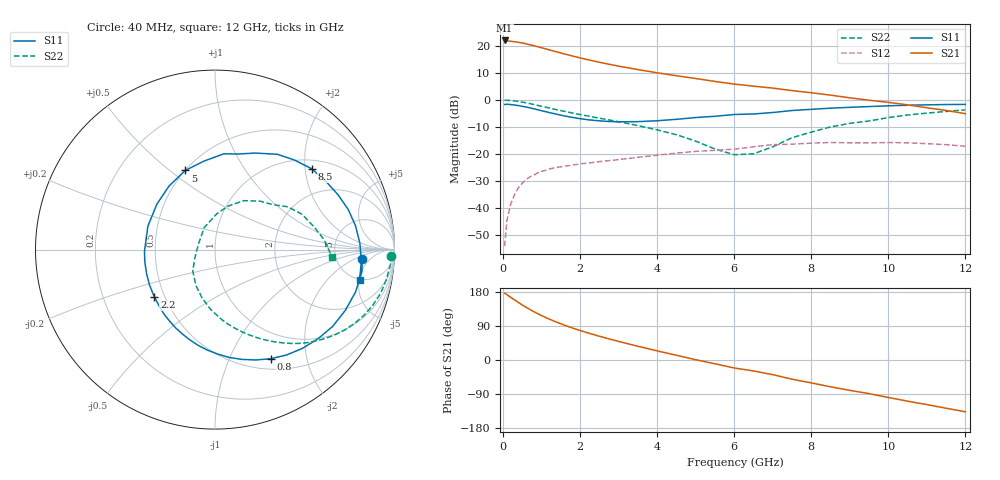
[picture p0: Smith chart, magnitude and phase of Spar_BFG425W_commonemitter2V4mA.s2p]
! Filename: 24bfg425.001
! BFG425W Field C1
! V1=8.240E-001V,V2=2.000E+000V, I1=5.227E-005A, I2=4.000E-003A
# GHz  S  MA  R 50
!  S11  S21  S12  S22
!Freq(GHz)  Mag  Ang  Mag  Ang  Mag  Ang  Mag  Ang
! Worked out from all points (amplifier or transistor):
!   44 points, 40 MHz to 12 GHz, reference 50 ohm
!   highest |S21| = 21.9 dB at 40 MHz (marker M1)
!   |S21| within 3 dB of that: start of sweep to 1.081 GHz
!   unconditionally stable (mu >= 1): 2.635 GHz to end of sweep
!   at 700 MHz: K = 0.29, MSG = 24.3 dB, |S12| = -28.4 dB
!   at 2.4 GHz: K = 0.93, MSG = 18.6 dB, |S12| = -23.0 dB
!   at 12 GHz: K = 1.54, MAG = 1.7 dB, |S12| = -17.1 dB
!   lowest NFmin = 1.00 dB at 900 GHz
!   S11 on the Smith chart (normalised r, x): 40 MHz: 9.30, -2.83; 800 MHz: 0.63, -1.44; 2.2 GHz: 0.44, -0.28; 5 GHz: 0.50, +0.57; 8.5 GHz: 1.22, +2.17; 12 GHz: 4.89, -5.09
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0.04  0.821 -3.5  12.43 176.4  0.002 74.1  0.983 -2.0
0.1  0.828 -8.4  12.17 172.4  0.006 86.0  0.981 -5.0
0.3  0.801 -25.0  11.78 158.6  0.018 74.9  0.954 -14.8
0.5  0.759 -40.9  11.19 145.0  0.029 65.7  0.907 -23.9
0.6  0.735 -48.5  10.77 138.9  0.034 61.4  0.879 -28.0
0.8  0.683 -62.9  9.945 127.6  0.041 54.1  0.819 -35.5
0.9  0.656 -69.6  9.544 122.3  0.045 50.9  0.789 -38.9
1.1  0.606 -82.5  8.725 112.5  0.05 45.3  0.733 -44.9
1.4  0.541 -100.2  7.632 99.5  0.057 38.7  0.655 -52.7
1.8  0.473 -122.0  6.43 84.5  0.063 32.3  0.571 -61.4
2.2  0.429 -141.9  5.493 71.6  0.068 27.7  0.503 -69.3
2.6  0.404 -160.8  4.761 59.9  0.074 23.9  0.445 -76.7
3  0.393 -178.6  4.18 49.0  0.079 20.5  0.394 -84.2
3.5  0.396 160.8  3.608 36.3  0.087 16.1  0.335 -94.0
4.5  0.437 125.9  2.783 12.5  0.104 6.0  0.227 -117.8
5  0.471 110.6  2.47 0.8  0.112 -0.9  0.173 -135.7
6  0.536 84.7  1.95 -21.1  0.123 -14.0  0.097 163.9
6.5  0.548 76.4  1.785 -28.9  0.136 -14.9  0.101 144.8
7.5  0.635 56.7  1.478 -50.6  0.152 -33.3  0.2 87.1
8.5  0.702 39.9  1.22 -70.8  0.163 -49.7  0.316 59.6
10.5  0.794 9.7  0.807 -108.6  0.161 -84.1  0.524 22.0
12  0.823 -11.8  0.554 -136.7  0.139 -114.3  0.653 -3.5
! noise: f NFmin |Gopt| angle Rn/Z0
900  1  0.28  11.7  0.24
2000  1.2  0.22  60.8  0.18
